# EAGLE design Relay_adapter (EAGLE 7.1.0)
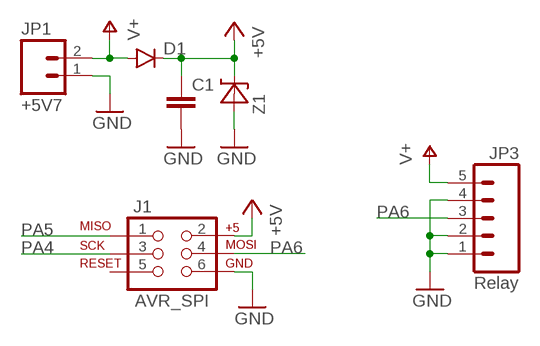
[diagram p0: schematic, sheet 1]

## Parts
C1  C-EUC1206  [C1206]
D1  DIODESMA  [SMA-DIODE]
J1  AVR_SPI  AVR_SPI_PRG_6PTH  [2X3]
JP1  +5V7  M02PTH  [1X02]
JP3  Relay  M05PTH  [1X05]
Z1  5V1  ZENER-SOD123SOD-123  [SOD123]

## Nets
+5V: C1.1 D1.C J1.2 Z1.C
GND: C1.2 J1.6 JP1.1 JP3.1 JP3.2 JP3.4 Z1.A
PA4: J1.3
PA5: J1.1
PA6: J1.4 JP3.3
V+: D1.A JP1.2 JP3.5
Unconnected: J1.5

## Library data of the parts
C1 = rcl:C-EU: CAPACITOR, European symbol
D1 = SparkFun-DiscreteSemi:DIODE: Diode
J1 = SparkFun-Connectors:AVR_SPI_PRG_6: AVR ISP 6 Pin This is the reduced ISP connector for AVR programming. Common on Arduino. This footprint will take up less PCB space and can be used with a 10-pin to 6-pin adapter such as SKU: BOB-08508 **Special note about "TEST_POINT" package. The stop mask is on the top side, so if you want your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
JP1 = SparkFun-Connectors:M02: Standard 2-pin 0.1" header. Use with
JP3 = SparkFun-Connectors:M05: Header 5 Standard 5-pin 0.1" header. Use with straight break away headers (SKU : PRT-00116), right angle break away headers (PRT-00553), swiss pins (PRT-00743), machine pins (PRT-00117), and female headers (PRT-00115). Molex polarized connector foot print use with SKU : PRT-08230 with associated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
Z1 = diode:ZENER-SOD123

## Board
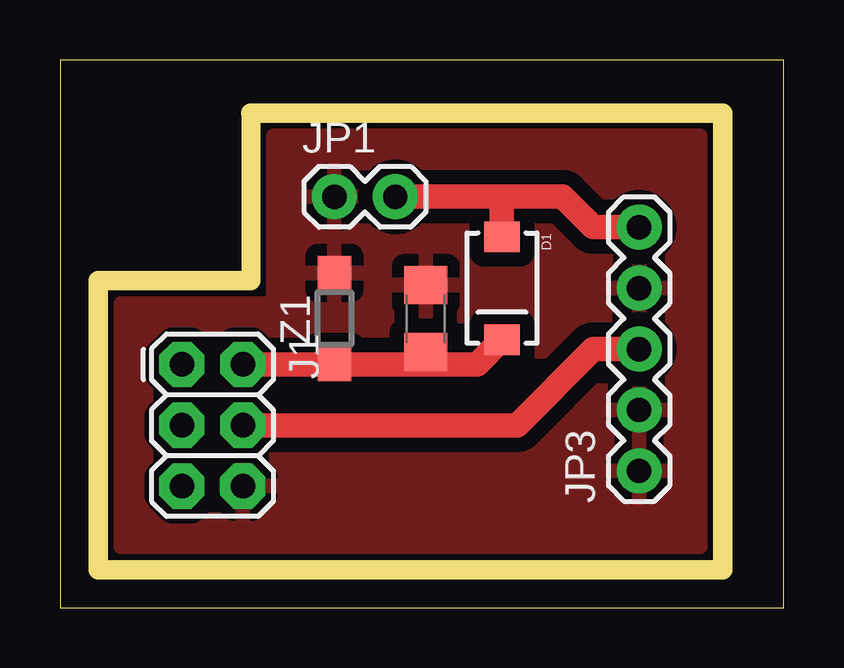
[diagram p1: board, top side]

Size 30.15 x 22.85 mm. Coordinates in mm from the lower left corner, seen from the top.
Outline: 0,0 30.15,0 30.15,22.85 0,22.85 0,0
Copper layers (1*16): Top 0.035mm / dielectric 1.5mm / Bottom 0.035mm
Design rules "default *": minimum track width 10mil, minimum drill 24mil, track to track 8mil, track to pad 8mil, pad to pad 8mil, via to via 8mil, smd to smd 8mil, copper to edge 40mil, drill to drill 8mil, minimum pad ring 10mil, minimum via ring 8mil, stop-mask expansion 4mil, vias tented up to drill 0mil, thermal gap 20mil
Milling: 6 lines

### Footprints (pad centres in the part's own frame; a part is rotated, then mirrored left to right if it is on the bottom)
C1206 = smd 1.6 x 1.8: 1 -1.4,0; 2 1.4,0
SMA-DIODE = smd 1.27 x 1.47: A -2.15,0; C 2.15,0
2X3 = drill 1.016 pad 1.88 octagon: 1 0,0; 2 0,2.54; 3 2.54,0; 4 2.54,2.54; 5 5.08,0; 6 5.08,2.54
1X02 = drill 1.016 pad 1.88: 1 0,0; 2 2.54,0
1X05 = drill 1.016 pad 1.88: 1 0,0; 2 2.54,0; 3 5.08,0; 4 7.62,0; 5 10.16,0
SOD123 = smd 1.4 x 1.4: A 1.9,0; C -1.9,0

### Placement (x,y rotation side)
C1  15.24,12.06 90 top
D1  18.41,13.34 270 top
J1  5.08,10.16 270 top
JP1  11.43,17.14 0 top
JP3  24.13,5.71 90 top
Z1  11.43,12.06 90 top

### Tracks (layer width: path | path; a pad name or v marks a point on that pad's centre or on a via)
+5V
  Top 1.016: J1.2 Z1.C | Z1.C 15.24,10.16 | Z1.C | C1.1 15.24,10.16 | 15.24,10.16 17.39,10.16 D1.C
GND
  pour Top (isolate 0.61): 2.54,12.7 8.89,12.7 8.89,19.68 26.67,19.68 26.67,2.54 2.54,2.54
PA6
  Top 1.016: J1.4 19.05,7.62 22.23,10.79 JP3.3
V+
  Top 1.016: JP1.2 18.41,17.14 | 18.41,17.14 20.95,17.14 22.23,15.88 JP3.5 | D1.A 18.41,17.14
